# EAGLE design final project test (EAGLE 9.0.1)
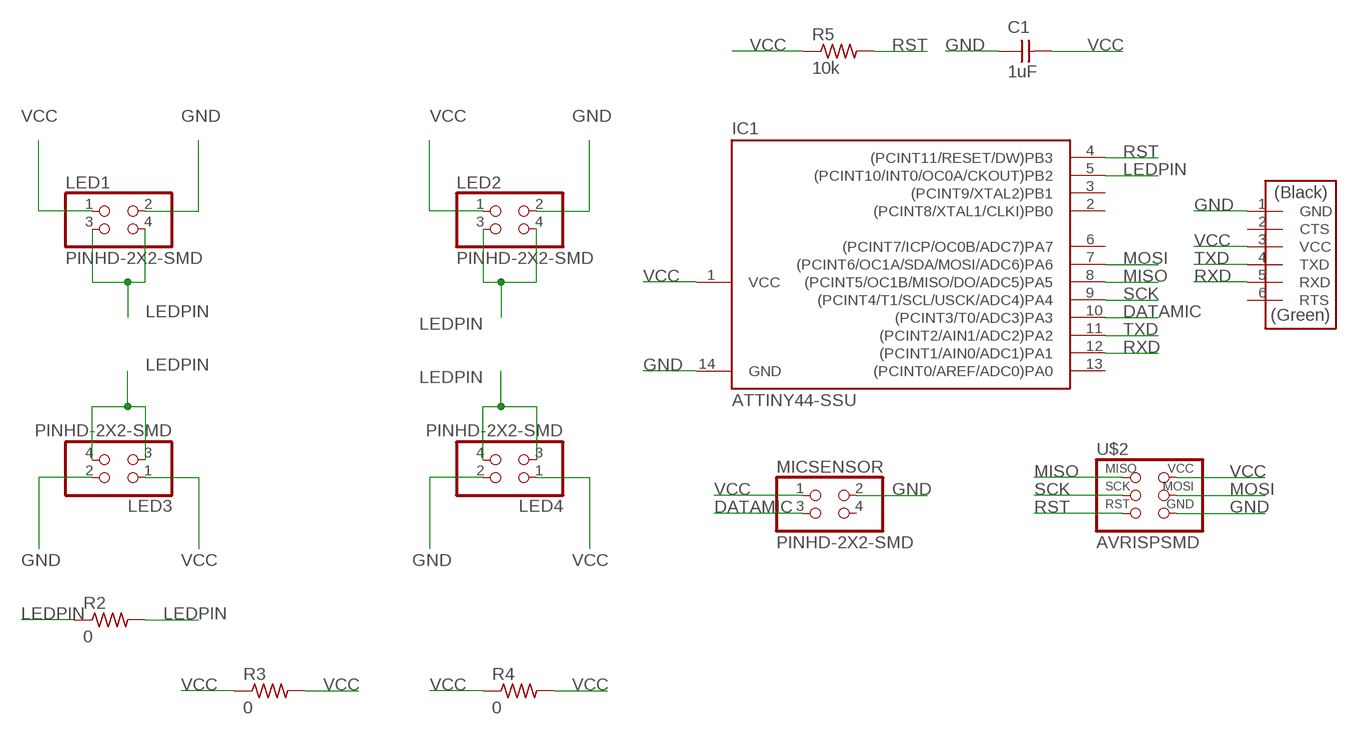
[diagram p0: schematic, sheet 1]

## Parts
C1  1uF  CAP-UNPOLARIZEDFAB  [C1206FAB]
IC1  ATTINY44-SSU  [SOIC14]
LED1  PINHD-2X2-SMD  [2X02SMD]
LED2  PINHD-2X2-SMD  [2X02SMD]
LED3  PINHD-2X2-SMD  [2X02SMD]
LED4  PINHD-2X2-SMD  [2X02SMD]
MICSENSOR  PINHD-2X2-SMD  [2X02SMD]
R2  0  RES-US1206FAB  [R1206FAB]
R3  0  RES-US1206FAB  [R1206FAB]
R4  0  RES-US1206FAB  [R1206FAB]
R5  10k  RES-US1206FAB  [R1206FAB]
U$2  AVRISPSMD  [2X03SMD]
U$6  FTDI-SMD-HEADER  [1X06SMD]

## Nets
DATAMIC: IC1.10((PCINT3/T0/ADC3)PA3) MICSENSOR.3
GND: C1.1 IC1.14(GND) LED1.2 LED2.2 LED3.2 LED4.2 MICSENSOR.2 U$2.6(GND) U$6.1(GND)
LEDPIN: IC1.5((PCINT10/INT0/OC0A/CKOUT)PB2) LED1.3 LED1.4 LED2.3 LED2.4 LED3.3 LED3.4 LED4.3 LED4.4 R2.1 R2.2
MISO: IC1.8((PCINT5/OC1B/MISO/DO/ADC5)PA5) U$2.1(MISO)
MOSI: IC1.7((PCINT6/OC1A/SDA/MOSI/ADC6)PA6) U$2.4(MOSI)
RST: IC1.4((PCINT11/RESET/DW)PB3) R5.2 U$2.5(RST)
RXD: IC1.12((PCINT1/AIN0/ADC1)PA1) U$6.5(RXD)
SCK: IC1.9((PCINT4/T1/SCL/USCK/ADC4)PA4) U$2.3(SCK)
TXD: IC1.11((PCINT2/AIN1/ADC2)PA2) U$6.4(TXD)
VCC: C1.2 IC1.1(VCC) LED1.1 LED2.1 LED3.1 LED4.1 MICSENSOR.1 R3.1 R3.2 R4.1 R4.2 R5.1 U$2.2(VCC) U$6.3(VCC)
Unconnected: IC1.2((PCINT8/XTAL1/CLKI)PB0) IC1.3((PCINT9/XTAL2)PB1) IC1.6((PCINT7/ICP/OC0B/ADC7)PA7) IC1.13((PCINT0/AREF/ADC0)PA0) MICSENSOR.4 U$6.2(CTS) U$6.6(RTS)

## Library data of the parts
C1 = fab:CAP-UNPOLARIZED
IC1 = fab:ATTINY44
LED1-LED4 MICSENSOR = fab:PINHD-2X2-SMD
R2-R5 = fab:RES-US: Resistor (US Symbol)
U$2 = fab:AVRISP
U$6 = fab:FTDI-SMD-HEADER

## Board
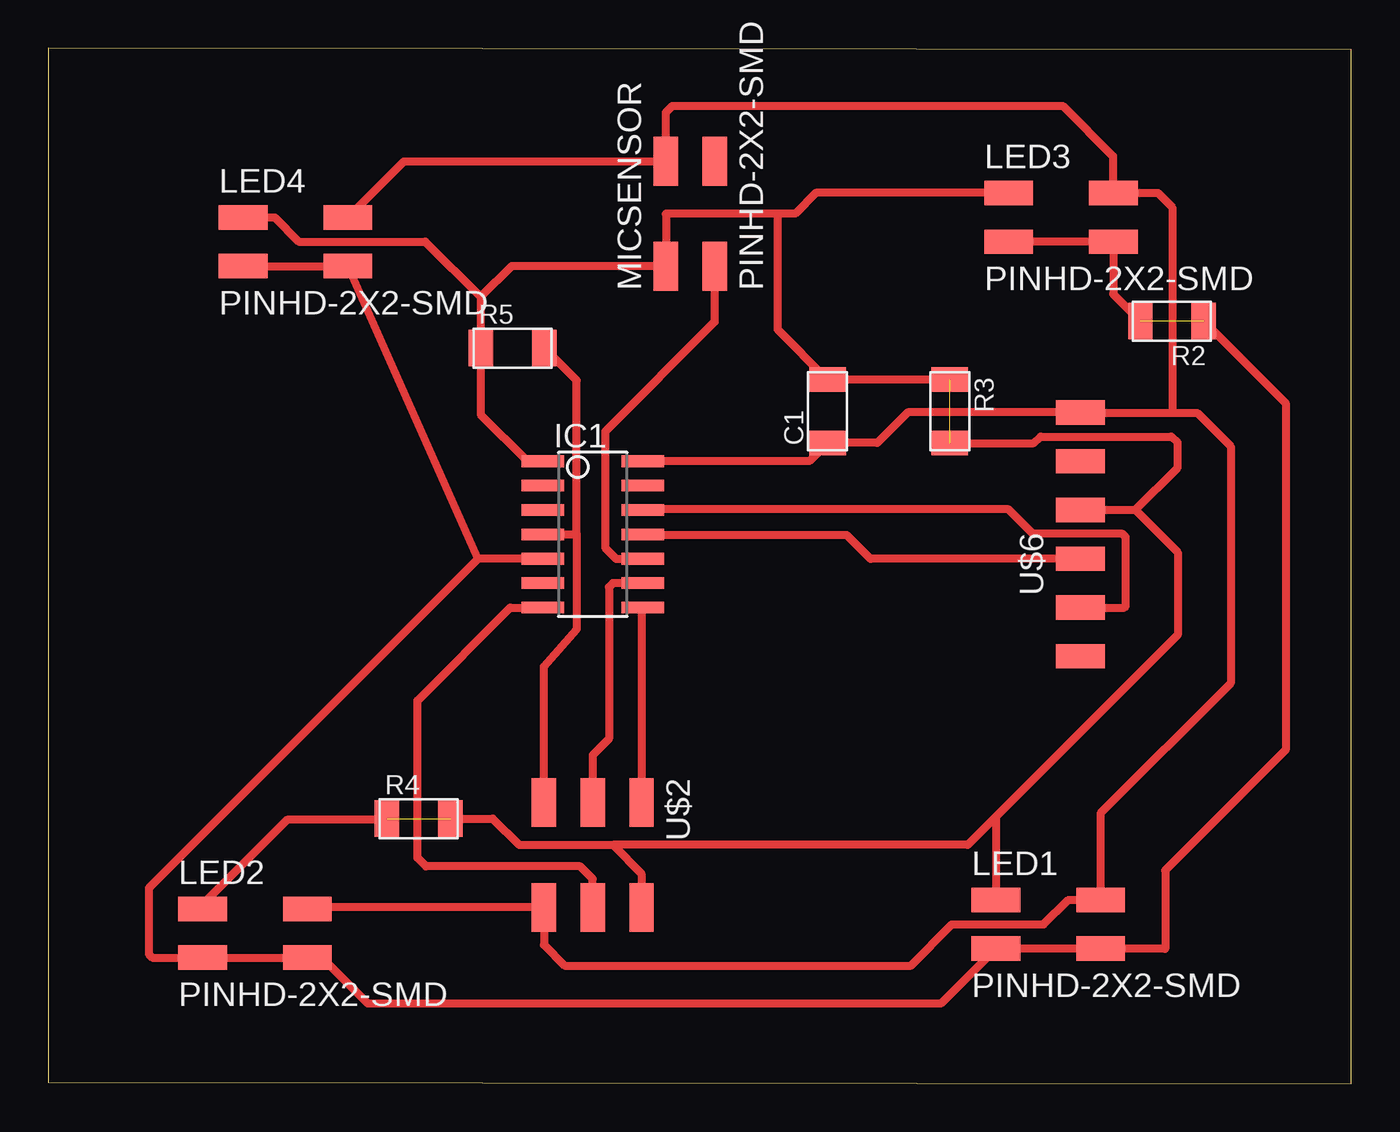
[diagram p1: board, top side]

Size 67.91 x 53.95 mm. Coordinates in mm from the lower left corner, seen from the top.
Outline: 0.02,0.09 67.91,0 67.89,53.86 0,53.95 0.02,0.09
Copper layers (1*16): Top 0.035mm / dielectric 1.5mm / Bottom 0.035mm
Design rules "default": minimum track width 6mil, minimum drill 0.35mm, track to track 6mil, track to pad 6mil, pad to pad 6mil, via to via 6mil, smd to smd 6mil, copper to edge 40mil, drill to drill 6mil, minimum pad ring 10mil, minimum via ring 8mil, stop-mask expansion 4mil, vias tented up to drill 0mil, thermal gap 10mil

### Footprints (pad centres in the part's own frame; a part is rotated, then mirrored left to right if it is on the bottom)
C1206FAB = smd 1.27 x 1.905: 1 -1.651,0; 2 1.651,0
SOIC14 = smd 0.61 x 2.21: 1 -3.81,-2.603; 2 -2.54,-2.603; 3 -1.27,-2.603; 4 0,-2.603; 5 1.27,-2.603; 6 2.54,-2.603; 7 3.81,-2.603; 8 3.81,2.603; 9 2.54,2.603; 10 1.27,2.603; 11 0,2.603; 12 -1.27,2.603; 13 -2.54,2.603; 14 -3.81,2.603
2X02SMD = smd 2.54 x 1.27: 1 -2.54,1.27; 2 2.92,1.27; 3 -2.54,-1.27; 4 2.92,-1.27
R1206FAB = smd 1.27 x 1.905: 1 -1.651,0; 2 1.651,0
2X03SMD = smd 2.54 x 1.27: 1 -2.54,2.54; 2 2.92,2.54; 3 -2.54,0; 4 2.92,0; 5 -2.54,-2.54; 6 2.92,-2.54
1X06SMD = smd 2.54 x 1.27: 1 0,6.35; 2 0,3.81; 3 0,1.27; 4 0,-1.27; 5 0,-3.81; 6 0,-6.35

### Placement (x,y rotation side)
C1  40.62,35.04 90 top
IC1  28.38,28.62 270 top
LED1  51.92,8.32 0 top
LED2  10.6,7.85 0 top
LED3  52.58,45.13 0 top
LED4  12.71,43.86 0 top
MICSENSOR  33.46,45.13 90 top
R2  58.56,39.72 180 top
R3  46.98,35.03 270 top
R4  19.32,13.82 0 top
R5  24.21,38.32 0 top
U$2  28.38,12.11 270 top
U$6  53.78,28.62 0 top

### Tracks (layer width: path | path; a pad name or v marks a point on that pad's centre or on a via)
DATAMIC
  Top 0.406: MICSENSOR.3 34.73,39.68 29.02,33.98 29.02,27.93 29.61,27.35 IC1.10
GND
  Top 0.406: 58.58,34.95 53.81,34.95 U$6.1 44.8,34.97 43.21,33.39 C1.1 39.67,32.43 IC1.14 | 58.58,34.95 59.88,34.95 61.62,33.2 61.62,20.87 54.84,14.09 LED1.2 53.17,9.59 51.87,8.32 47.09,8.32 44.97,6.16 26.92,6.16 25.84,7.24 U$2.6 25.83,9.21 13.6,9.21 LED2.2 | LED4.2 18.55,48.05 MICSENSOR.2 32.19,50.6 32.53,50.94 52.87,50.94 55.48,48.33 55.48,46.42 LED3.2 57.83,46.4 58.58,45.65 58.58,34.95
LEDPIN  (1 unrouted)
  Top 0.406: LED3.3 LED3.4 55.5,41.13 R2.2 | LED4.3 LED4.4 22.41,27.35 | 25.77,27.34 IC1.5 22.41,27.35 | 22.41,27.35 5.26,10.2 5.26,6.76 5.44,6.58 LED2.3 LED2.4 14.28,6.58 16.68,4.19 46.52,4.19 LED1.3 LED1.4 58.21,7.04 58.21,11.13 64.48,17.39 64.48,35.46 R2.1
MISO
  Top 0.406: IC1.8 30.92,24.75 U$2.1
MOSI
  Top 0.406: U$2.4 28.38,10.68 27.73,11.33 19.69,11.33 19.25,11.77 19.25,19.97 24.08,24.8 25.77,24.8 IC1.7
RST
  Top 0.406: IC1.4 27.16,28.62 27.54,28.63 | 27.54,28.63 27.54,23.69 25.83,21.73 25.83,14.67 U$2.5 | 27.54,28.63 27.54,36.64 R5.2
RXD
  Top 0.406: IC1.12 31.02,29.93 50.04,29.93 51.32,28.64 55.99,28.64 56.15,28.48 56.15,27.18 56.15,24.89 56.07,24.81 U$6.5
SCK
  Top 0.406: IC1.9 29.44,26.08 29.23,25.87 29.23,17.97 28.38,17.13 U$2.3
TXD
  Top 0.406: U$6.4 42.86,27.35 41.63,28.59 31.02,28.59 IC1.11
VCC  (2 unrouted)
  Top 0.406: LED3.1 40.01,46.4 38.94,45.33 38.01,45.33 | 38.01,45.33 32.22,45.33 32.19,45.3 MICSENSOR.1 | 32.13,42.53 MICSENSOR.1 | MICSENSOR.1 24.15,42.59 22.55,40.99 | 22.55,40.99 22.55,38.33 R5.1 22.56,34.87 22.55,34.86 24.98,32.43 IC1.1 | 38.01,45.33 38.02,45.32 38.02,39.29 C1.2 40.63,36.68 R3.1 47,36.69 | U$6.3 56.65,29.89 | 56.65,29.89 58.86,27.69 58.86,23.39 49.38,13.91 | R4.1 17.6,13.76 12.46,13.76 8.06,9.35 LED2.1 | R4.2 23.18,13.82 24.55,12.45 29.43,12.45 | U$2.2 30.92,10.96 29.43,12.45 | R3.2 51.35,33.38 51.71,33.71 58.53,33.71 58.86,33.41 58.86,32.1 56.65,29.89 | LED4.1 11.82,45.13 13.06,43.87 19.65,43.87 22.55,40.99 | 49.38,13.91 49.38,9.68 | 49.38,9.68 LED1.1 | 49.26,9.56 49.38,9.68 | 49.38,13.91 47.92,12.45 29.43,12.45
